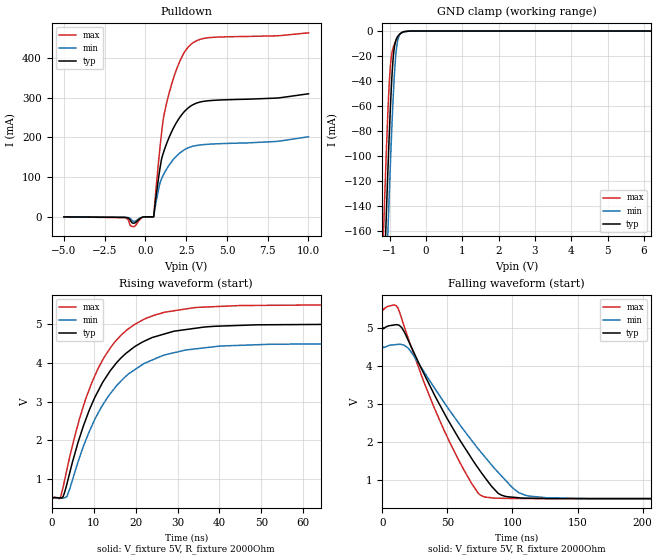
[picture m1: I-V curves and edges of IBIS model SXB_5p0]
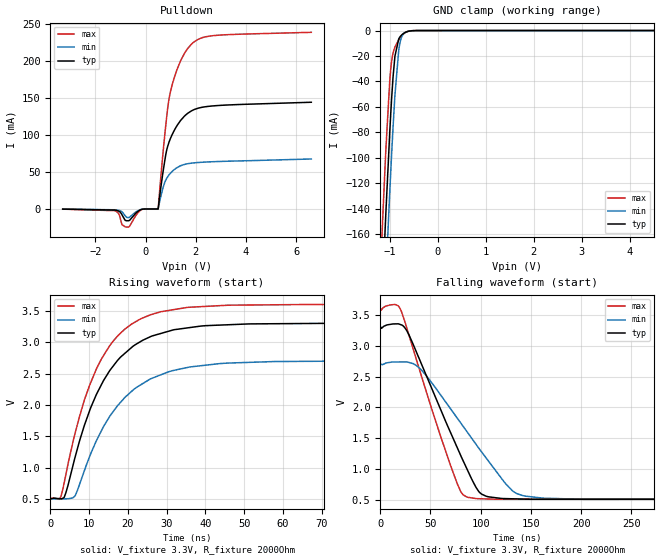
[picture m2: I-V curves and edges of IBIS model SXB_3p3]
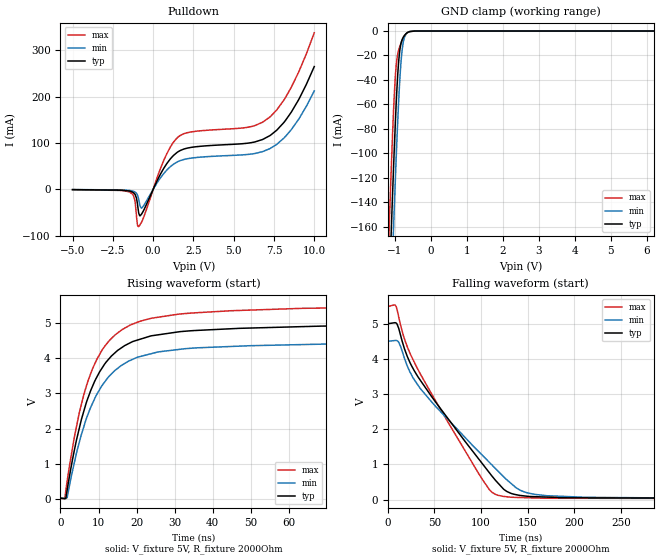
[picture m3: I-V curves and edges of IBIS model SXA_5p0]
|Texas Instruments Incorporated
| Level-Translating I2C Bus Repeater
| Marketing part#   Digital Voltage Range   Package-type   #pins
| TCA9517DGKR   2.7V - 5.5V   MSOP   8
| TCA9517DSGR   2.7V - 5.5V   QFN   8
[IBIS Ver]   4.1
[File name]   tca9517.ibs
[File Rev]   1.0
[Date]   2/20/2013
[Source]
| Texas Instruments Incorporated.
| Analog-eLab Design Center, HPA
| 12500 TI Blvd
| Dallas, TX -75243
| e-mail: elab_scm_ibis@list.ti.com
[Notes]   Revision History:
| Rev 1.0: 2/20/2013
| - Initial version of the model
| - Model generated from simulations in TISPICE
| - C_comp although listed in numerical order of value are
|   obtained from varying PVT conditions. For PVT conditions for
|   each specific value refer the buffer description under
|   respective [Model]. IBIS model user is responsible for using
|   appropriate C_comp to simulate for Signal Integrity.
| - Warnings regarding combined Non-monotonicity of various models have been
|   reviewd and considered minor and can be ignored.
| - Model names with a trailing _0p9v contains the model for
|   0.9V operation.Model names with a trailing _3p3 contains the model
|   for 3.3V operation.Model names with a trailing _5p0 contains the model
|   for 5.0V operation.
[Disclaimer]
| This model is designed as an aid for customers of Texas Instruments.
| TI and its licensors and suppliers make no warranties, either expressed
| or implied, with respect to this  model, including the warranties of
| merchantability or fitness for a particular purpose. The model is
| provided solely on an "as is" basis. The entire risk as to its quality
| and performance is with the customer.
[Copyright]
 (C) Copyright 2013 Texas Instruments Incorporated.All rights reserved.
|   TPA9517
[Component]   TPA9517
[Manufacturer]   TI
[Package]
|   typ   min   max
R_pkg   0.0933   0.0850   0.110
L_pkg   2.139nH   2.002nH   2.414nH
C_pkg   0.409pF   0.393pF   0.419pF
[Pin]  signal_name   model_name   R_pin   L_pin   C_pin
1   VCCA   POWER   0.09509   2.17891nH   0.39356pF
2   SCLA   SXA   0.08551   2.01249nH   0.41943pF
3   SDAA   SXA   0.08546   2.01168nH   0.41843pF
4   GND   GND   0.11001   2.41491nH   0.40705pF
5   EN   EN   0.10454   2.31962nH   0.40281pF
6   SDAB   SXB   0.08546   2.00264nH   0.41903pF
7   SCLB   SXB   0.08551   2.00349nH   0.41916pF
8   VCCB   POWER   0.0951   2.17119nH   0.39331pF
|   Model Selectors
[Model Selector]  SXA
SXA_5p0   Buffer in 5V operation
SXA_3p3   Buffer in 3.3V operation
SXA_0p9   Buffer in 0.9V operation
[Model Selector]  SXB
SXB_5p0   Buffer in 5V operation
SXB_3p3   Buffer in 3.3V operation
[Model Selector]  EN
EN_5p0   Buffer in 5V operation
EN_3p3   Buffer in 3.3V operation
| Models and submodels in the file (7): SXB_5p0 (I/O_open_drain), SXB_3p3 (I/O_open_drain), SXA_5p0 (I/O_open_drain), SXA_3p3 (I/O_open_drain), SXA_0p9 (I/O_open_drain), EN_3p3 (Input), EN_5p0 (Input)
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|   Model
|   Model
[Model]   SXB_5p0
Model_type   I/O_open_drain
Polarity   Non-Inverting
Enable   Active-Low
Vinl = 1.5
Vinh = 2.1
Vmeas = 2.5
Vref = 5
Cref = 1pF
Rref = 2000
|   typ   min   max
C_comp   2.401pF   2.193pF   2.846pF
[Voltage Range]   5   4.5   5.5
[Temperature Range]   25   85   -40
[Pullup Reference]   5   4.5   5.5
[Pulldown Reference]   0   0   0
[Power Clamp Reference]   5   4.5   5.5
[GND Clamp Reference]   0   0   0
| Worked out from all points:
|   slope of the pulldown table from 0 to 0.75 V, typ, clamps not added: 9.18 ohm
|   GND clamp passes 1 mA (typ) near -0.64 V on its own axis
|   falling waveform, V_fixture 5V, R_fixture 2000Ohm: 20-80 % time 44.1ns typ, 51.4ns min, 36.7ns max; typ from 5 V to 0.512 V
|   rising waveform, V_fixture 5V, R_fixture 2000Ohm: 20-80 % time 11.4ns typ, 12.3ns min, 10.6ns max; typ from 0.511 V to 5 V
[Pulldown]
|   Voltage   I(typ)   I(min)   I(max)
-5V       -93.89uA   -85.31uA   -112.1uA
-1.25V    -1.344mA   -1.022mA   -2.084mA
-725mV    -15.94mA   -11.6mA    -24.56mA
-185mV    -854.2uA   -640uA     -1.274mA
505mV     56.85uA    96.71uA    37.59uA
895mV     123.1mA    85.76mA    175.8mA
1.165V    169.4mA    110.7mA    261.9mA
1.645V    217.7mA    141.1mA    339.2mA
2.005V    244.4mA    157.1mA    382mA
2.845V    280.8mA    177mA      436.2mA
4V        292.8mA    183.2mA    451.6mA
10V       309.9mA    201.7mA    463.4mA
[GND Clamp]
|   Voltage   I(typ)   I(min)   I(max)
-5V       -3.969A    -4.012A    -3.926A
-1.16V    -209.2mA   -260.8mA   -156.9mA
-1.115V   -170.1mA   -221.2mA   -118.8mA
-1.085V   -144.7mA   -195.4mA   -94.72mA
-1.04V    -108.2mA   -157.5mA   -61.83mA
-980mV    -64.18mA   -109.7mA   -29.47mA
-920mV    -29.97mA   -66.69mA   -15.62mA
-875mV    -14.77mA   -39.83mA   -11.26mA
-830mV    -7.85mA    -20.15mA   -8.115mA
-770mV    -4.125mA   -6.733mA   -4.805mA
-620mV    -669.5uA   -654.4uA   -597.9uA
10V       0A         0A         0A
[POWER Clamp]
|   Voltage   I(typ)   I(min)   I(max)
-5V       0A         0A         0A
-4.97V    0A         0A         0A
-4.955V   0A         0A         0A
10V       0A         0A         0A
[Ramp]
R_load = 2000
|   typ   min   max
dV/dt_r   2.69352/1.14108e-08   2.39369/1.2289e-08   2.9934/1.05997e-08
dV/dt_f   2.6927/4.41089e-08   2.39278/5.14518e-08   2.99282/3.67385e-08
[Falling Waveform]
V_fixture = 5V
V_fixture_min = 4.5V
V_fixture_max = 5.5V
R_fixture = 2000Ohm
C_fixture = 0F
|   Time   V(typ)   V(min)   V(max)
0s        5V         4.5V       5.5V
11.91ns   5.076V     4.563V     5.525V
20.79ns   4.611V     4.43V      4.642V
46.85ns   2.806V     3.075V     2.357V
67.15ns   1.649V     2.112V     1V
77.9ns    1.113V     1.648V     565.1mV
89.61ns   641.1mV    1.183V     523.9mV
104.8ns   536.4mV    670.2mV    515.1mV
126.5ns   516.6mV    536mV      514.9mV
500ns     512.2mV    512mV      512mV
[Rising Waveform]
V_fixture = 5V
V_fixture_min = 4.5V
V_fixture_max = 5.5V
R_fixture = 2000Ohm
C_fixture = 0F
|   Time   V(typ)   V(min)   V(max)
0s        510.9mV    510.6mV    511.1mV
2.107ns   512.4mV    509.9mV    535.4mV
3.583ns   856.9mV    543.7mV    1.223V
8.146ns   2.545V     2.01V      3.084V
11.03ns   3.267V     2.698V     3.85V
14.22ns   3.836V     3.241V     4.427V
21.75ns   4.547V     3.967V     5.114V
33.87ns   4.891V     4.359V     5.427V
74.09ns   4.999V     4.499V     5.499V
500ns     5V         4.5V       5.5V
|   Model
[Model]   SXB_3p3
Model_type   I/O_open_drain
Polarity   Non-Inverting
Enable   Active-Low
Vinl = 0.99
Vinh = 2.31
Vmeas = 1.65
Vref = 3.3
Cref = 1pF
Rref = 2000
|   typ   min   max
C_comp   2.401pF   2.193pF   2.846pF
[Voltage Range]   3.3   2.7   3.6
[Temperature Range]   25   85   -40
[Pullup Reference]   3.3   2.7   3.6
[Pulldown Reference]   0   0   0
[Power Clamp Reference]   3.3   2.7   3.6
[GND Clamp Reference]   -0   -0   0
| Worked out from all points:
|   slope of the pulldown table from 0 to 0.495 V, typ, clamps not added: 7.81 kohm
|   GND clamp passes 1 mA (typ) near -0.65 V on its own axis
|   falling waveform, V_fixture 3.3V, R_fixture 2000Ohm: 20-80 % time 44.4ns typ, 58.7ns min, 36.4ns max; typ from 3.3 V to 0.506 V
|   rising waveform, V_fixture 3.3V, R_fixture 2000Ohm: 20-80 % time 11.8ns typ, 13.1ns min, 11ns max; typ from 0.505 V to 3.3 V
[Pulldown]
|   Voltage   I(typ)   I(min)   I(max)
-3.3V     -166.1uA   -150.2uA   -200.3uA
-1.231V   -1.432mA   -1.081mA   -2.262mA
-933.9mV  -8.229mA   -3.864mA   -21.26mA
-745.8mV  -15.92mA   -11.41mA   -24.55mA
-171.6mV  -691uA     -521.9uA   -1.014mA
501.6mV   99.71uA    434uA      53.22uA
798.6mV   72.23mA    38.57mA    111.2mA
986.7mV   95.07mA    48.27mA    157.9mA
1.403V    120mA      58.58mA    200.9mA
1.957V    134.7mA    62.46mA    226.5mA
2.888V    139.9mA    64.18mA    234.9mA
6.6V      144.3mA    67.62mA    238.8mA
[GND Clamp]
|   Voltage   I(typ)   I(min)   I(max)
-3.3V     -2.284A    -2.33A     -2.238A
-1.191V   -236.9mA   -288.7mA   -184.3mA
-1.142V   -193.2mA   -244.7mA   -141.3mA
-1.092V   -150.8mA   -201.6mA   -100.5mA
-1.082V   -142.5mA   -193.1mA   -92.7mA
-1.003V   -80.39mA   -127.7mA   -39.84mA
-983.4mV  -66.48mA   -112.3mA   -30.79mA
-933.9mV  -36.64mA   -76.05mA   -17.58mA
-894.3mV  -20.08mA   -50.62mA   -12.89mA
-795.3mV  -5.332mA   -10.78mA   -6.088mA
-656.7mV  -1.13mA    -1.109mA   -1.119mA
6.6V      0A         0A         0A
[POWER Clamp]
|   Voltage   I(typ)   I(min)   I(max)
-3.3V     0A         0A         0A
-3.28V    0A         0A         0A
-3.27V    0A         0A         0A
6.6V      0A         0A         0A
[Ramp]
R_load = 2000
|   typ   min   max
dV/dt_r   1.6768/1.184e-08   1.31787/1.30913e-08   1.85659/1.09701e-08
dV/dt_f   1.67654/4.42938e-08   1.3176/5.8414e-08   1.85641/3.63534e-08
[Falling Waveform]
V_fixture = 3.3V
V_fixture_min = 2.7V
V_fixture_max = 3.6V
R_fixture = 2000Ohm
C_fixture = 0F
|   Time   V(typ)   V(min)   V(max)
0s        3.3V       2.7V       3.6V
20.43ns   3.344V     2.738V     3.582V
39.1ns    2.777V     2.637V     2.609V
69.13ns   1.621V     1.995V     1.094V
79.77ns   1.228V     1.753V     640.6mV
85.78ns   1.016V     1.616V     545.3mV
100.9ns   588.7mV    1.275V     512.7mV
131.7ns   512.7mV    640.5mV    506mV
144.5ns   507.2mV    555.8mV    506mV
500ns     505.8mV    504mV      506mV
[Rising Waveform]
V_fixture = 3.3V
V_fixture_min = 2.7V
V_fixture_max = 3.6V
R_fixture = 2000Ohm
C_fixture = 0F
|   Time   V(typ)   V(min)   V(max)
0s        505.4mV    503.7mV    505.7mV
2.697ns   505.5mV    505.4mV    536.3mV
4.014ns   600.3mV    506.2mV    889.7mV
6.313ns   1.149V     545.2mV    1.527V
10.09ns   1.899V     1.169V     2.306V
15.27ns   2.541V     1.812V     2.939V
23.81ns   3.03V      2.34V      3.385V
35.25ns   3.227V     2.596V     3.553V
79.28ns   3.3V       2.7V       3.599V
500ns     3.3V       2.7V       3.6V
|   Model
[Model]   SXA_5p0
Model_type   I/O_open_drain
Polarity   Non-Inverting
Enable   Active-Low
Vinl = 1.5
Vinh = 2.1
Vmeas = 2.5
Vref = 5
Cref = 1pF
Rref = 2000
|   typ   min   max
C_comp   1.711pF   1.625pF   1.872pF
[Voltage Range]   5   4.5   5.5
[Temperature Range]   25   85   -40
[Pullup Reference]   5   4.5   5.5
[Pulldown Reference]   0   0   0
[Power Clamp Reference]   5   4.5   5.5
[GND Clamp Reference]   0   -0   0
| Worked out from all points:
|   slope of the pulldown table from 0 to 0.75 V, typ, clamps not added: 14.9 ohm
|   GND clamp passes 1 mA (typ) near -0.64 V on its own axis
|   falling waveform, V_fixture 5V, R_fixture 2000Ohm: 20-80 % time 79.4ns typ, 89.6ns min, 68.9ns max; typ from 5 V to 0.032 V
|   rising waveform, V_fixture 5V, R_fixture 2000Ohm: 20-80 % time 10ns typ, 10.5ns min, 9.54ns max; typ from 0.031 V to 5 V
[Pulldown]
|   Voltage   I(typ)   I(min)   I(max)
-5V       -360.2uA   -230.6uA   -484.3uA
-1.475V   -3.355mA   -2.119mA   -5.057mA
-1.13V    -10.16mA   -5.359mA   -23.64mA
-980mV    -28.96mA   -11.51mA   -74.59mA
-905mV    -48.58mA   -19.74mA   -80.17mA
-695mV    -51.93mA   -39.76mA   -69.03mA
595mV     41.76mA    31.42mA    57.25mA
1.48V     79.76mA    59.1mA     111mA
6.1V      101.1mA    76.5mA     135.9mA
7.24V     116.1mA    88.08mA    156.2mA
8.575V    166.9mA    129.1mA    220.6mA
10V       265.3mA    212.6mA    338.2mA
[GND Clamp]
|   Voltage   I(typ)   I(min)   I(max)
-5V       -3.969A    -4.012A    -3.926A
-1.25V    -291.3mA   -343.5mA   -238.2mA
-1.16V    -210.8mA   -262.7mA   -158.3mA
-1.115V   -172mA     -223.3mA   -120.5mA
-1.07V    -134.5mA   -185mA     -85.31mA
-1.04V    -110.7mA   -160.1mA   -64.25mA
-980mV    -67.22mA   -112.7mA   -32.47mA
-890mV    -21.92mA   -51.98mA   -14.69mA
-830mV    -9.647mA   -23.88mA   -9.68mA
-770mV    -4.998mA   -8.892mA   -5.799mA
-620mV    -747uA     -747.6uA   -670.3uA
10V       0A         0A         0A
[POWER Clamp]
|   Voltage   I(typ)   I(min)   I(max)
-5V       0A         0A         0A
-4.97V    0A         0A         0A
-4.955V   0A         0A         0A
10V       0A         0A         0A
[Ramp]
R_load = 2000
|   typ   min   max
dV/dt_r   2.98123/9.97181e-09   2.67781/1.05124e-08   3.28469/9.53291e-09
dV/dt_f   2.98084/7.92588e-08   2.67679/8.93848e-08   3.28459/6.87849e-08
[Falling Waveform]
V_fixture = 5V
V_fixture_min = 4.5V
V_fixture_max = 5.5V
R_fixture = 2000Ohm
C_fixture = 0F
|   Time   V(typ)   V(min)   V(max)
0s        5V         4.5V       5.5V
8.481ns   5.023V     4.525V     5.508V
11.65ns   4.868V     4.474V     5.194V
18.68ns   4.225V     3.953V     4.499V
31.92ns   3.507V     3.27V      3.717V
97.8ns    1.145V     1.357V     727.3mV
115.8ns   539.7mV    875.4mV    145.9mV
142.7ns   116.2mV    258.6mV    58.29mV
170.7ns   71.46mV    110mV      38.02mV
500ns     31.93mV    38.68mV    25.69mV
[Rising Waveform]
V_fixture = 5V
V_fixture_min = 4.5V
V_fixture_max = 5.5V
R_fixture = 2000Ohm
C_fixture = 0F
|   Time   V(typ)   V(min)   V(max)
0s        31.25mV    36.92mV    25.49mV
1.131ns   18.78mV    27.43mV    20.9mV
1.763ns   264.5mV    49.23mV    515.3mV
3.688ns   1.407V     1.057V     1.78V
6.1ns     2.48V      2.043V     2.948V
10.84ns   3.7V       3.206V     4.206V
18.89ns   4.46V      3.957V     4.954V
30.73ns   4.733V     4.236V     5.235V
119.2ns   4.961V     4.448V     5.48V
500ns     5V         4.5V       5.5V
